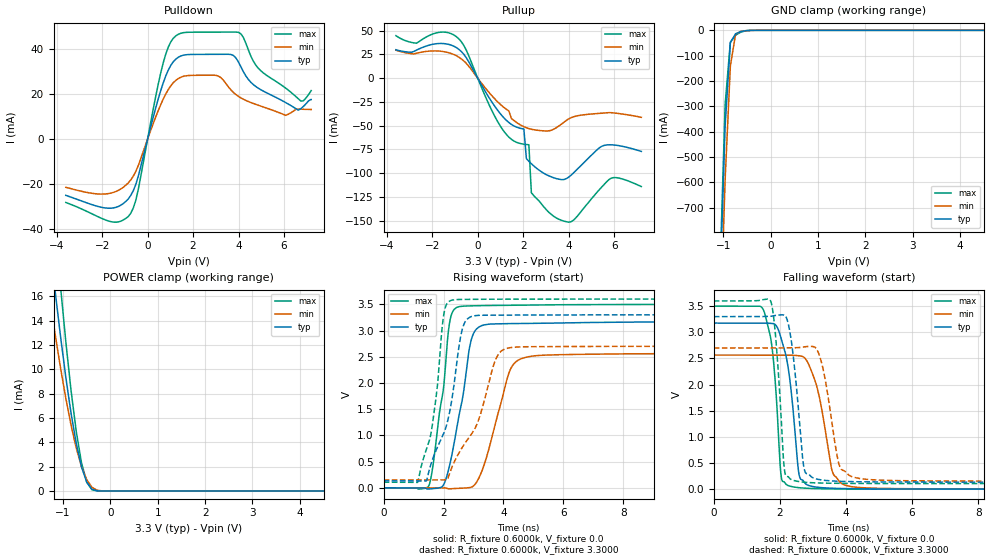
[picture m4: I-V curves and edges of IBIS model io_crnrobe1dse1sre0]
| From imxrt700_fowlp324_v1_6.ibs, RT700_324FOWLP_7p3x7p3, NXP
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[Model] io_crnrobe1dse1sre0
|   Model io_crnrobe1dse1sre0
| This model was characterised for following simulation conditions:
| External (pad) voltage:
|   - Typ: 3.3V,   - Min: 2.7V,   - Max: 3.6V
| Library cells for typ/min/max conditions are connected as defined below:
|  PAD_IO - External Pad
|  ipp_do - Core Input
|  ipp_obe - Output Buffer Enable
|  ASRCN3V3[3] - NC
|  ASRCN3V3[4] - NC
|  ASRCP3V3[4] - NC
|  REFAPBIAS3V3 - gnde
|  REFBAMPL3V3 - vdd1v8
|  REFCAMPH3V3 - vdd1v8
|  REFDNBIAS3V3 - vdd1v8
|  REFH3V3 - REFH3V3
|  REFL3V3 - REFL3V3
|  gnde - gnde
|  ipp_dse - vdd
|  ipp_ina235_3v - NC
|  ipp_ina40_3v - NC
|  ipp_ina_mux - NC
|  ipp_ind - NC
|  ipp_ind_1p8v - NC
|  ipp_ind_3v - NC
|  ipp_sre - gnde
|  vdd - vdd
|  vdd1v8 - vdd1v8
|  vdda - vdde3v3
|  vdde3v3 - vdde3v3
| All other pins connected to ground
Model_type I/O
Polarity   Non-Inverting
Enable   Active-High
Vinl =   0.9900V
Vinh =   2.3100V
Vmeas =  1.6500V
Cref =   15.0000pF
Rref =   0.6000k
Vref =   0.0V
C_comp   4.0038pF   3.8208pF   4.1229pF
|C_comp_pullup   0.5150pF   0.5958pF   0.4948pF
|C_comp_pulldown   2.0815pF   2.1737pF   1.8626pF
[Model Spec]
| variable   typ   min   max
Vinh   2.3100V   NA   NA
Vinl   0.9900V   NA   NA
Vref   0.0V   0.0V   0.0V
Cref   15.0000pF   15.0000pF   15.0000pF
Rref   0.6000k   0.6000k   0.6000k
[Receiver Thresholds]
Vcross_high  =   0.0V
Vcross_low  =   0.0V
Vdiff_ac  =   0.0V
Vdiff_dc  =   0.0V
Tdiffslew_ac  =   0.0S
[Temperature Range]   25.0000   0.1250k   -40.0000
[Voltage Range]   3.3000V   2.7000V   3.6000V
[Pullup Reference]   3.3000V   2.7000V   3.6000V
[Pulldown Reference]   0.0V   0.0V   0.0V
[POWER Clamp Reference]   3.3000V   2.7000V   3.6000V
[GND Clamp Reference]   0.0V   0.0V   0.0V
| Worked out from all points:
|   slope of the pulldown table from 0 to 0.495 V, typ, clamps not added: 26.5 ohm
|   slope of the pullup table from 0 to 0.495 V, typ, clamps not added: 24.3 ohm
|   GND clamp passes 1 mA (typ) near -0.49 V on its own axis
|   POWER clamp passes 1 mA (typ) near -0.52 V on its own axis
|   rising waveform, R_fixture 0.6000k, V_fixture 0.0: 20-80 % time 549ps typ, 711ps min, 417ps max; typ from 0 V to 3.18 V
|   rising waveform, R_fixture 0.6000k, V_fixture 3.3000: 20-80 % time 718ps typ, 1.09ns min, 456ps max; typ from 0.133 V to 3.3 V
|   falling waveform, R_fixture 0.6000k, V_fixture 0.0: 20-80 % time 329ps typ, 452ps min, 241ps max; typ from 3.18 V to 0 V
|   falling waveform, R_fixture 0.6000k, V_fixture 3.3000: 20-80 % time 280ps typ, 383ps min, 211ps max; typ from 3.3 V to 0.133 V
[Pulldown]
|Voltage   I(typ)   I(min)   I(max)
-3.6V     -24.99mA   -21.42mA   -28.15mA
-1.73V    -30.7mA    -24.22mA   -36.35mA
-740mV    -24.98mA   -18.14mA   -32.92mA
-410mV    -16.5mA    -11.77mA   -22.36mA
690mV     24.98mA    17.78mA    33.89mA
1.35V     36.27mA    26.82mA    46.47mA
3.11V     37.58mA    27.95mA    47.42mA
3.99V     34.3mA     18.95mA    47.34mA
5.09V     21.27mA    14.22mA    29.34mA
6.08V     16.14mA    10.5mA     22.54mA
6.74V     13.43mA    13.23mA    16.85mA
7.2V      17.5mA     13.09mA    21.48mA
[Pullup]
|Voltage   I(typ)   I(min)   I(max)
-3.6V     30.01mA    29.47mA    44.8mA
-830mV    30.4mA     22.17mA    41.43mA
820mV     -31.95mA   -23.5mA    -43.27mA
1.7V      -51.43mA   -46.46mA   -67.41mA
2.03V     -53.47mA   -51.07mA   -69.49mA
2.14V     -84.67mA   -52.15mA   -69.82mA
2.25V     -87.44mA   -53.03mA   -70.06mA
2.36V     -90.02mA   -53.72mA   -120.6mA
3.46V     -105.7mA   -52.08mA   -147.2mA
4.23V     -99.3mA    -40.51mA   -149.1mA
5.88V     -70.12mA   -36.3mA    -105.2mA
7.2V      -77.09mA   -41.15mA   -114.1mA
[GND_clamp]
|Voltage   I(typ)   I(min)   I(max)
-3.6V     -19.67A    -19.55A    -20.65A
-1.07V    -1.013A    -1.224A    -956.3mA
-960mV    -377.1mA   -587.4mA   -291.7mA
-850mV    -48.2mA    -140.8mA   -46.94mA
-740mV    -13.57mA   -15.62mA   -19.22mA
-630mV    -5.136mA   -4.37mA    -7.235mA
-520mV    -1.276mA   -1.53mA    -1.554mA
-300mV    -4.356uA   -32.48uA   -995.7nA
7.2V      0A         0A         0A
[POWER_clamp]
|Voltage   I(typ)   I(min)   I(max)
-3.6V     102.7mA    81.65mA    131.1mA
-1.38V    23.95mA    18.52mA    31.78mA
-1.27V    20.01mA    15.56mA    26.56mA
-1.16V    16.22mA    12.73mA    21.52mA
-1.05V    12.64mA    10.07mA    16.71mA
-830mV    6.384mA    5.406mA    8.254mA
-720mV    3.9mA      3.518mA    4.888mA
-610mV    1.982mA    2.008mA    2.327mA
-500mV    727.2uA    927.8uA    733.5uA
-390mV    144.5uA    302.5uA    95.96uA
-170mV    198.4nA    4.047uA    20.3nA
7.2V      0A         0A         0A
[Ramp]
| variable   typ   min   max
dV/dt_r  1.9062/0.5490n   1.5390/0.7105n   2.1005/0.4169n
dV/dt_f  1.9001/0.2799n   1.5294/0.3832n   2.0958/0.2115n
R_load = 0.6000k
[Rising Waveform]
R_fixture= 0.6000k
V_fixture= 0.0
V_fixture_min= 0.0
V_fixture_max= 0.0
|time   V(typ)   V(min)   V(max)
0s        57.42nV    1.433uV    55.99nV
1.523ns   -21.29mV   -492.7uV   57.33mV
2ns       56.4mV     -597.4uV   1.899V
2.209ns   441mV      -18.88mV   3.17V
2.616ns   1.645V     -8.613mV   3.463V
2.882ns   2.712V     5.378mV    3.47V
3.101ns   3.028V     104.2mV    3.473V
4.239ns   3.132V     2.265V     3.482V
5.129ns   3.137V     2.522V     3.489V
60ns      3.177V     2.565V     3.501V
[Rising Waveform]
R_fixture= 0.6000k
V_fixture= 3.3000
V_fixture_min= 2.7000
V_fixture_max= 3.6000
|time   V(typ)   V(min)   V(max)
0s        133.2mV    151mV      107mV
1.141ns   132.4mV    151mV      110.4mV
1.603ns   490.2mV    150.6mV    1.109V
2.033ns   1.074V     150.7mV    3.379V
2.331ns   1.883V     462.1mV    3.585V
2.568ns   2.873V     716.4mV    3.592V
2.778ns   3.21V      901.1mV    3.594V
3.784ns   3.293V     2.498V     3.597V
4.422ns   3.296V     2.684V     3.598V
60ns      3.3V       2.7V       3.6V
[Falling Waveform]
R_fixture= 0.6000k
V_fixture= 0.0
V_fixture_min= 0.0
V_fixture_max= 0.0
|time   V(typ)   V(min)   V(max)
0s        3.177V     2.565V     3.501V
1.482ns   3.178V     2.565V     3.453V
1.747ns   3.171V     2.564V     2.794V
1.923ns   3.094V     2.565V     1.454V
2.058ns   2.844V     2.566V     183.3mV
2.614ns   207.6mV    2.549V     26.15mV
3.114ns   38.35mV    1.973V     10.21mV
3.61ns    16.92mV    297.4mV    4.805mV
4.409ns   7.172mV    31.67mV    1.692mV
60ns      1.139uV    2.252uV    983.1nV
[Falling Waveform]
R_fixture= 0.6000k
V_fixture= 3.3000
V_fixture_min= 2.7000
V_fixture_max= 3.6000
|time   V(typ)   V(min)   V(max)
0s        3.3V       2.7V       3.6V
1.72ns    3.306V     2.7V       3.6V
1.88ns    3.324V     2.699V     2.866V
2.179ns   3.303V     2.702V     259.1mV
2.395ns   2.605V     2.704V     171.5mV
2.731ns   405.9mV    2.722V     133.6mV
3.218ns   180.5mV    2.521V     117.4mV
3.826ns   149.8mV    413.3mV    111mV
4.722ns   139.3mV    183.2mV    108.3mV
60ns      133.2mV    151mV      107mV
